ORGANIZATION_BLOCK MAIN:OB1
TITLE=

BEGIN
NETWORK 1
LD I0.0
O I0.1
A T36
O M0.0
AN T35
= M0.0

NETWORK 2
LDN M0.0
= Q0.4

NETWORK 3
LD M0.0
TON T32 +300

NETWORK 4
LD M0.0
LDN T32
O T34
ALD
= Q0.3

NETWORK 5
LD M0.0
A T32
= Q0.2

NETWORK 6
LD Q0.2
TON T33 +100

NETWORK 7
LD Q0.2
AN T33
= Q0.1

NETWORK 8
LD M0.0
A T33
TON T34 +100

NETWORK 9
LD M0.0
LDN T32
O T33
ALD
ON M0.0
= Q0.0

NETWORK 10
LD M0.0
A T34
TON T35 +30

NETWORK 11
LD Q0.4
TON T36 +10

END_ORGANIZATION_BLOCK

